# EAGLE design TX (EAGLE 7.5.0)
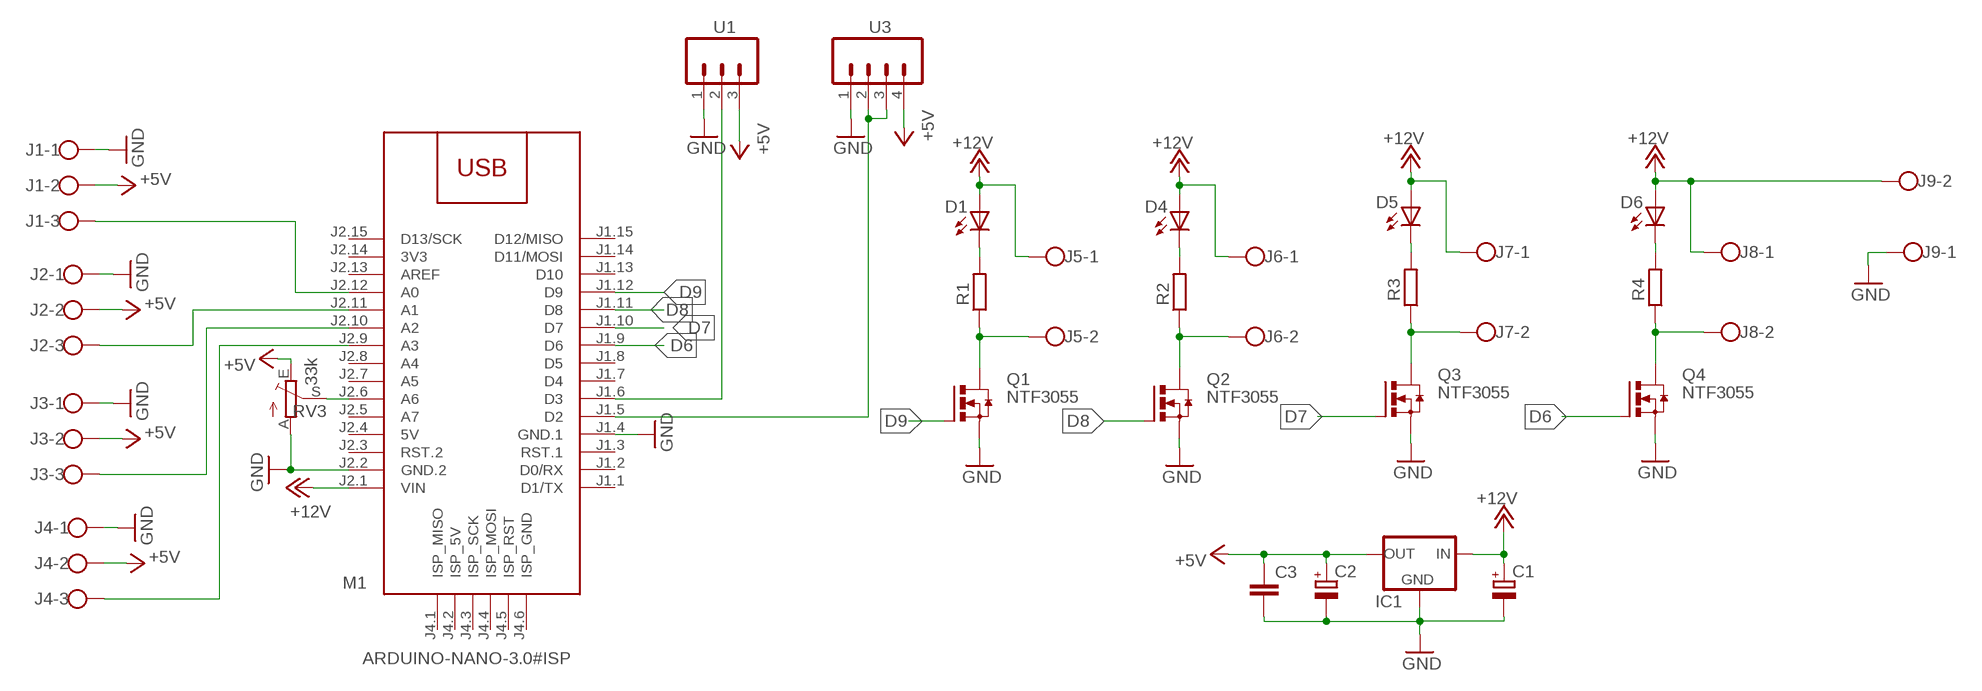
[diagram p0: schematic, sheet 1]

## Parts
C1  CPOL-EUE2.5-6  [E2,5-6]
C2  CPOL-EUE2.5-6  [E2,5-6]
C3  C-EUC1206  [C1206]
D1  LED5MM  [LED5MM]
D4  LED5MM  [LED5MM]
D5  LED5MM  [LED5MM]
D6  LED5MM  [LED5MM]
IC1  78XXL  [78XXL]
J1  W237-103  [W237-103]
J2  W237-103  [W237-103]
J3  W237-103  [W237-103]
J4  W237-103  [W237-103]
J5  W237-102  [W237-102]
J6  W237-102  [W237-102]
J7  W237-102  [W237-102]
J8  W237-102  [W237-102]
J9  W237-102  [W237-102]
M1  ARDUINO-NANO-3.0#ISP  [ARDUINO-NANO-3.0#ISP]
Q1  NTF3055  N-HEXFET_SOT323-  [SOT223]
Q2  NTF3055  N-HEXFET_SOT323-  [SOT223]
Q3  NTF3055  N-HEXFET_SOT323-  [SOT223]
Q4  NTF3055  N-HEXFET_SOT323-  [SOT223]
R1  R-EU_R1206  [R1206]
R2  R-EU_R1206  [R1206]
R3  R-EU_R1206  [R1206]
R4  R-EU_R1206  [R1206]
RV3  33k  TRIM_EU-CA6V  [CA6V]
U1  M03  [03P]
U3  M04  [04P]

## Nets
+5V: C2.+ C3.1 IC1.OUT J1.2 J2.2 J3.2 J4.2 RV3.E U1.3 U3.4
+12V: C1.+ D1.A D4.A D5.A D6.A IC1.IN J5.1 J6.1 J7.1 J8.1 J9.2 M1.J2.1(VIN)
D6: M1.J1.9(D6) Q4.1(G)
D7: M1.J1.10(D7) Q3.1(G)
D8: M1.J1.11(D8) Q2.1(G)
D9: M1.J1.12(D9) Q1.1(G)
GND: C1.- C2.- C3.2 IC1.GND J1.1 J2.1 J3.1 J4.1 J9.1 M1.J1.4(GND.1) M1.J2.2(GND.2) Q1.3(S) Q2.3(S) Q3.3(S) Q4.3(S) RV3.A U1.1 U3.1
N$1: M1.J1.6(D3) U1.2
N$2: M1.J1.5(D2) U3.2 U3.3
N$3: J5.2 Q1.4(D) R1.1
N$4: D1.K(C) R1.2
N$5: J7.2 Q3.4(D) R3.1
N$6: J6.2 Q2.4(D) R2.1
N$7: D4.K(C) R2.2
N$8: D5.K(C) R3.2
N$9: J8.2 Q4.4(D) R4.1
N$10: D6.K(C) R4.2
N$11: J1.3 M1.J2.12(A0)
N$12: J2.3 M1.J2.11(A1)
N$13: J3.3 M1.J2.10(A2)
N$14: J4.3 M1.J2.9(A3)
N$15: M1.J2.6(A6) RV3.S
Unconnected: M1.J1.1(D1/TX) M1.J1.2(D0/RX) M1.J1.3(RST.1) M1.J1.7(D4) M1.J1.8(D5) M1.J1.13(D10) M1.J1.14(D11/MOSI) M1.J1.15(D12/MISO) M1.J2.3(RST.2) M1.J2.5(A7) M1.J2.7(A5) M1.J2.8(A4) M1.J2.13(AREF) M1.J2.15(D13/SCK) M1.J4.1(ISP_MISO) M1.J4.2(ISP_5V) M1.J4.3(ISP_SCK) M1.J4.4(ISP_MOSI) M1.J4.5(ISP_RST) M1.J4.6(ISP_GND)

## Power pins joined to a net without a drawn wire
3V3: M1.J2.14(3V3)
5V: M1.J2.4(5V)

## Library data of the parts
C1 C2 = rcl:CPOL-EU: POLARIZED CAPACITOR, European symbol
C3 = rcl:C-EU: CAPACITOR, European symbol
D1 D4-D6 = led:LED: LED
IC1 = v-reg:78XXL: VOLTAGE REGULATOR
J1-J4 = con-wago-500:W237-103: WAGO SCREW CLAMP; MPN: 237-103; OC_FARNELL: unknown; OC_NEWARK: 18M7116
J5-J9 = con-wago-500:W237-102: WAGO SCREW CLAMP; MPN: 237-102; OC_FARNELL: unknown; OC_NEWARK: 70K9898
M1 = diy-modules:ARDUINO-NANO-3.0#ISP: Arduino Nano 3.0 (and compatible devices) with ISP pads More details available here: https://www.arduino.cc/en/Main/ArduinoBoardNano Click here to find device on ebay.com
Q1-Q4 = transistor-power:N-HEXFET_?-*: HEXFET® Power MOSFET
R1-R4 = rcl:R-EU_: RESISTOR, European symbol
RV3 = pot:TRIM_EU-: POTENTIOMETER
U1 = con-amp-quick:M03: AMP QUICK CONNECTOR; OC_FARNELL: unknown; OC_NEWARK: unknown
U3 = con-amp-quick:M04: AMP QUICK CONNECTOR; OC_FARNELL: unknown; OC_NEWARK: unknown

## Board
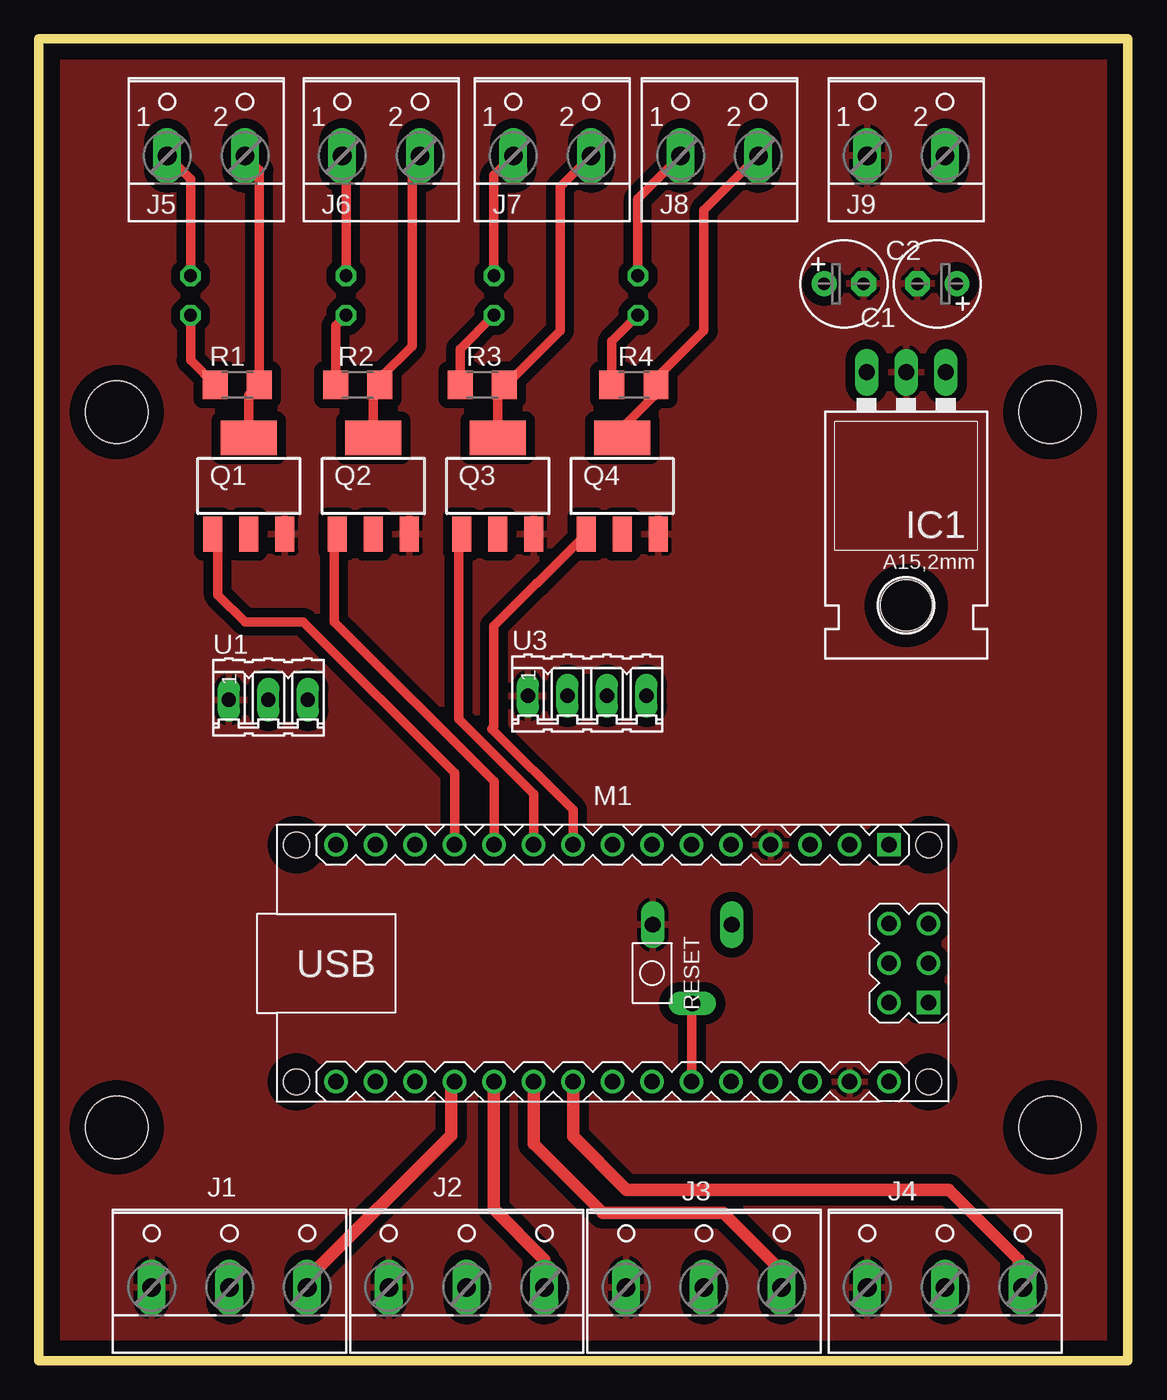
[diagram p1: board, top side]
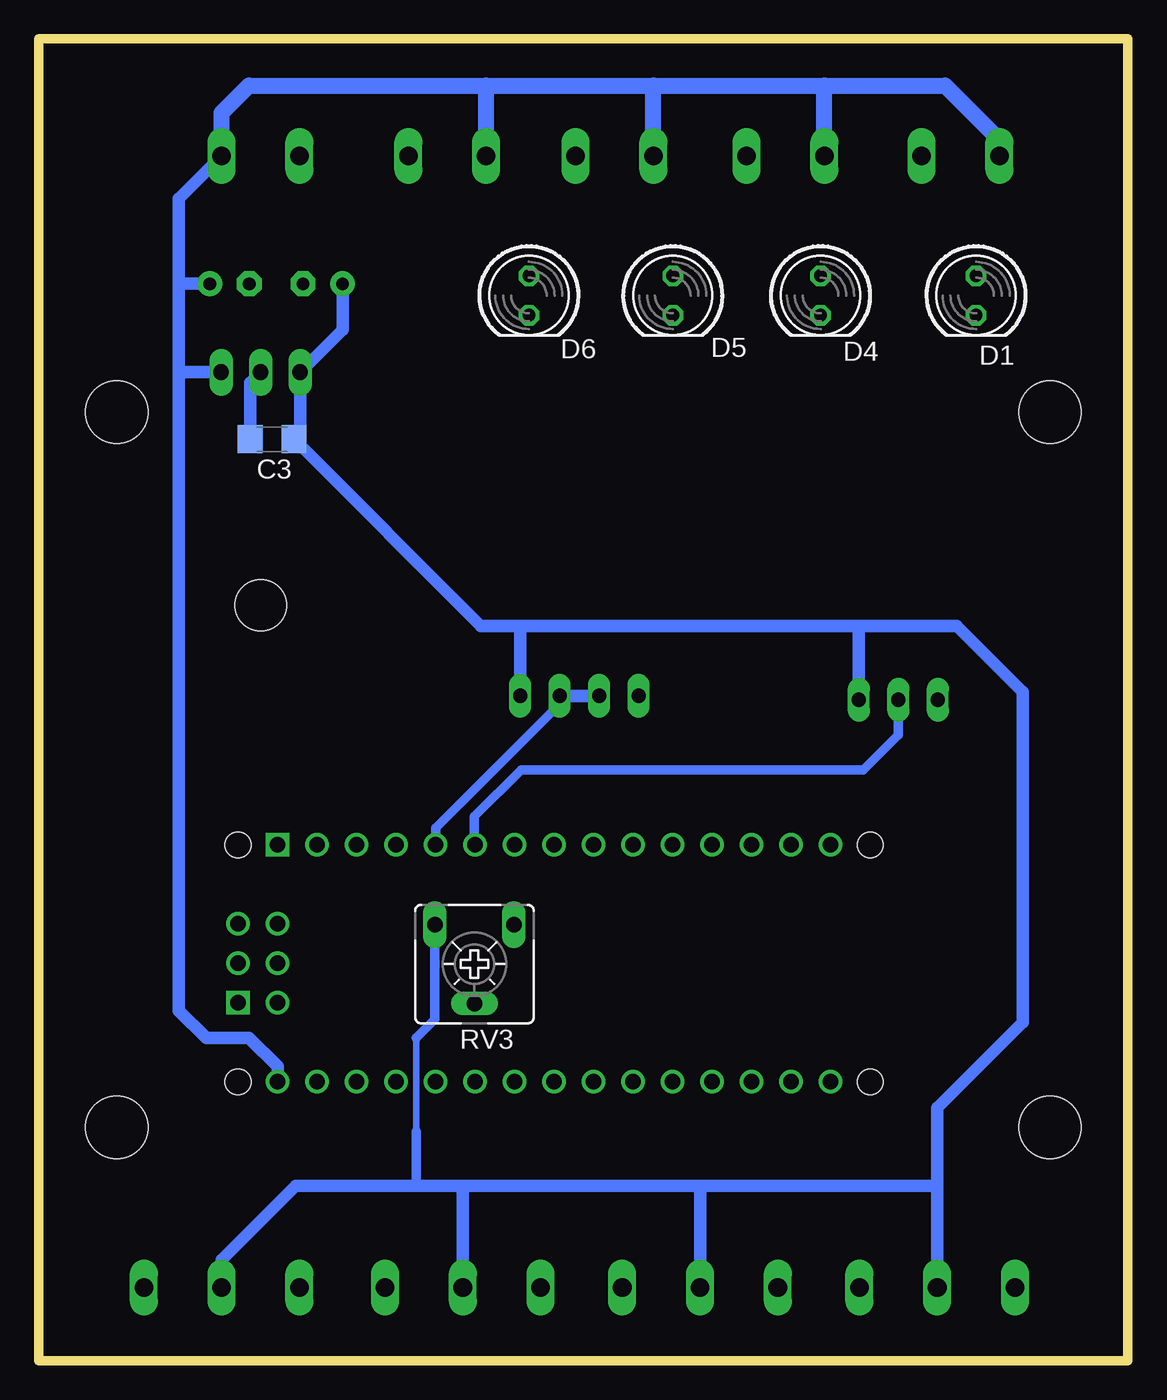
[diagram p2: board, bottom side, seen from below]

Size 70 x 85 mm. Coordinates in mm from the lower left corner, seen from the top.
Outline: 0,0 70,0 70,85 0,85 0,0
Copper layers (1*16): Top 0.035mm / dielectric 1.5mm / Bottom 0.035mm
Design rules "default": minimum track width 10mil, minimum drill 24mil, track to track 8mil, track to pad 8mil, pad to pad 8mil, via to via 8mil, smd to smd 8mil, copper to edge 40mil, drill to drill 8mil, minimum pad ring 10mil, minimum via ring 8mil, stop-mask expansion 4mil, vias tented up to drill 0mil, thermal gap 10mil
Holes 4 mm at 65,15 5,15 5,61 65,61

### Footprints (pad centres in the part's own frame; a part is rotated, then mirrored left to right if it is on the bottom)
E2,5-6 = drill 0.813 pad 1.6: + -1.27,0 | drill 0.813 pad 1.6 octagon: - 1.27,0
C1206 = smd 1.6 x 1.8: 1 -1.4,0; 2 1.4,0
LED5MM = drill 0.813 octagon: A -1.27,0; K 1.27,0
78XXL = drill 1.016 long: GND 0,-3.81; IN -2.54,-3.81; OUT 2.54,-3.81 | hole 3.302: 0,11.176
W237-103 = drill 1.194 long: 1 -5,-1.29; 2 0,-1.29; 3 5,-1.29
W237-102 = drill 1.194 long: 1 -2.5,-1.27; 2 2.5,-1.27
ARDUINO-NANO-3.0#ISP = drill 1 square: J1.1 17.78,7.62; J4.1 20.32,-2.54 | drill 1: J1.2 15.24,7.62; J1.3 12.7,7.62; J1.4 10.16,7.62; J1.5 7.62,7.62; J1.6 5.08,7.62; J1.7 2.54,7.62; J1.8 0,7.62; J1.9 -2.54,7.62; J1.10 -5.08,7.62; J1.11 -7.62,7.62; J1.12 -10.16,7.62; J1.13 -12.7,7.62; J1.14 -15.24,7.62; J1.15 -17.78,7.62; J2.1 17.78,-7.62; J2.2 15.24,-7.62; J2.3 12.7,-7.62; J2.4 10.16,-7.62; J2.5 7.62,-7.62; J2.6 5.08,-7.62; J2.7 2.54,-7.62; J2.8 0,-7.62; J2.9 -2.54,-7.62; J2.10 -5.08,-7.62; J2.11 -7.62,-7.62; J2.12 -10.16,-7.62; J2.13 -12.7,-7.62; J2.14 -15.24,-7.62; J2.15 -17.78,-7.62; J4.2 17.78,-2.54; J4.3 20.32,0; J4.4 17.78,0; J4.5 20.32,2.54; J4.6 17.78,2.54 | hole 1.651: -20.32,7.62; -20.32,-7.62; 20.32,-7.62; 20.32,7.62
SOT223 = smd 1.219 x 2.235: 1 -2.311,-3.099; 2 0,-3.099; 3 2.311,-3.099 | smd 3.6 x 2.2: 4 0,3.099
R1206 = smd 1.6 x 1.803: 1 -1.422,0; 2 1.422,0
CA6V = drill 1.016 long: A -2.54,-2.54; E 2.54,-2.54; S 0,2.54
03P = drill 0.914 long: 1 -2.54,0; 2 0,0; 3 2.54,0
04P = drill 0.914 long: 1 -3.81,0; 2 -1.27,0; 3 1.27,0; 4 3.81,0

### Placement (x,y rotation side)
C1  57.75,69.25 180 top
C2  51.75,69.25 0 top
C3  55,59.25 180 bottom
D1  9.75,68.5 270 bottom
D4  19.75,68.5 270 bottom
D5  29.25,68.5 270 bottom
D6  38.5,68.5 270 bottom
IC1  55.75,59.75 180 top
J1  12.25,6 0 top
J2  27.5,6 0 top
J3  42.75,6 0 top
J4  58.25,6 0 top
J5  10.75,78.75 0 top
J6  22,78.75 0 top
J7  33,78.75 0 top
J8  43.75,78.75 0 top
J9  55.75,78.75 0 top
M1  36.88,25.55 0 top
Q1  13.5,56.25 0 top
Q2  21.5,56.25 0 top
Q3  29.5,56.25 0 top
Q4  37.5,56.25 0 top
R1  12.75,62.75 180 top
R2  20.5,62.75 180 top
R3  28.5,62.75 180 top
R4  38.25,62.75 180 top
RV3  42,25.5 180 bottom
U1  14.75,42.5 0 top
U3  35.25,42.75 0 top

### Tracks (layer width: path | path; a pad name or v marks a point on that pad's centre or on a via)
+5V
  Bottom 0.406: 45.75,20.75 45.75,14.75
  Bottom 0.61: RV3.E 44.54,21.96 45.75,20.75 | 45.75,14.75 45.75,11.25
  Bottom 0.813: C2.+ 50.48,66.29 IC1.OUT 53.21,59.64 C3.1 41.6,47.25 39.25,47.25 | 17.5,47.25 11,47.25 6.75,43 6.75,21.75 12.25,16.25 12.25,11 | 17.5,47.25 39.25,47.25 | U3.4 39.06,47.06 39.25,47.25 | J1.2 12.25,11 | U1.3 17.29,47.04 17.5,47.25 | J4.2 58.25,6.5 53.5,11.25 45.75,11.25 42.5,11.25 | 42.5,11.25 27.25,11.25 | 27.25,11.25 12.5,11.25 12.25,11 | J3.2 42.75,11 42.5,11.25 | J2.2 27.5,11 27.25,11.25
+12V
  Top 0.61: D1.A 9.75,75.98 J5.1 | D4.A 19.75,77.23 J6.1 | D5.A 29.25,76.23 J7.1 | D6.A 38.5,74.73 J8.1
  Bottom 0.813: 59,69.23 C1.+ 60.75,69.25 61,69 | M1.J2.1 54.66,18.91 56.5,20.75 59.25,20.75 61,22.5 61,63.25 | 61,63.25 61,69 | 61,69 61,74.73 J9.2 | IC1.IN 60.69,63.56 61,63.25
  Bottom 1.016: J6.1 19.5,82 | 19.5,82 11.75,82 8.5,78.75 8.5,77.73 J5.1 | J7.1 30.5,82 | 30.5,82 19.5,82 | J8.1 41.25,82 | 41.25,82 30.5,82 | J9.2 58.25,80.25 56.5,82 41.25,82
D6
  Top 0.61: M1.J1.9 34.34,35.41 29.12,40.62 29.25,40.75 29.25,47.25 32,50 32.04,50 Q4.1
D7
  Top 0.61: M1.J1.10 31.8,36.45 27,41.25 27,52.96 Q3.1
D8
  Top 0.61: M1.J1.11 29.26,37.24 19,47.5 19,52.96 Q2.1
D9
  Top 0.61: M1.J1.12 26.72,37.78 17,47.5 13.25,47.5 11.5,49.25 11.5,52.84 Q1.1
GND
  Bottom 0.813: C3.2 56.4,62.91 IC1.GND
  pour Top (isolate 0.6): 1.25,84.25 69.5,84.25 69.5,0.75 1.25,0.75
N$1
  Bottom 0.61: U1.2 14.75,40.25 17,38 39,38 42,35 42,33.21 M1.J1.6
N$2
  Bottom 0.61: U3.3 36.52,42.23 44.5,34.25 M1.J1.5
  Bottom 0.813: U3.3 U3.2
N$3
  Top 0.61: Q1.4 13.5,62.08 R1.1 14.17,76.56 J5.2
N$4
  Top 0.61: D1.K 9.75,64.33 R1.2
N$5
  Top 0.61: Q3.4 29.5,62.33 R3.1 30,62.75 33.5,66.25 33.5,75.48 J7.2
N$6
  Top 0.61: Q2.4 21.5,62.33 R2.1 21.92,63.17 24,65.25 24,76.98 J6.2
N$7
  Top 0.61: R2.2 19.08,66.56 D4.K
N$8
  Top 0.61: R3.2 27.08,65.06 D5.K
N$9
  Top 0.61: Q4.4 37.5,60 39.5,62 39.5,62.58 R4.1 39.67,63.17 42.75,66.25 42.75,73.98 J8.2
N$10
  Top 0.61: R4.2 36.83,65.56 D6.K
N$11
  Top 0.813: J1.3 17.25,5.25 26.5,14.5 26.5,17.71 M1.J2.12
N$12
  Top 0.813: J2.3 32.5,6.5 29.25,9.75 M1.J2.11
N$13
  Top 0.813: M1.J2.10 31.8,13.95 36.25,9.5 44,9.5 47.75,5.75 J3.3
N$14
  Top 0.813: M1.J2.9 34.34,14.41 37.75,11 58.5,11 63,6.5 63,4.96 J4.3
N$15
  Top 0.61: RV3.S 41.96,22.96 M1.J2.6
